FUNCTION "DIVE" : VOID
TITLE =
VERSION : 0.1


VAR_TEMP
  zero : BOOL ;
END_VAR
BEGIN
NETWORK
TITLE =Produzione in corso
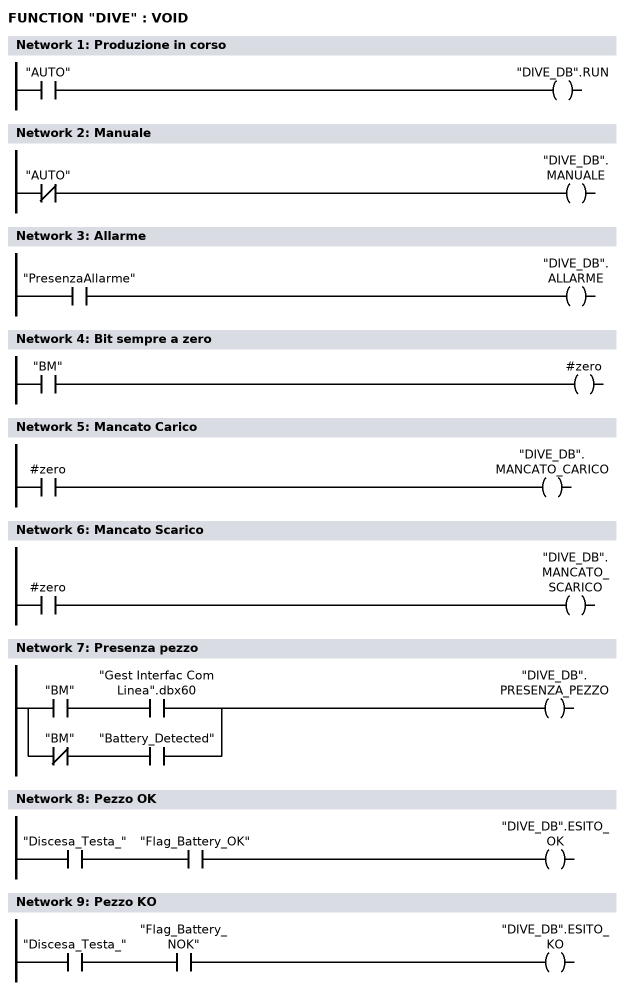
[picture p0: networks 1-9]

      U     "AUTO";
      =     "DIVE_DB".RUN;
NETWORK
TITLE =Manuale

      UN    "AUTO";
      =     "DIVE_DB".MANUALE;
NETWORK
TITLE =Allarme

      U     "PresenzaAllarme";
      =     "DIVE_DB".ALLARME;
NETWORK
TITLE =Bit sempre a zero

      U     "BM";
      =     #zero;
NETWORK
TITLE =Mancato Carico

      U     #zero;
      =     "DIVE_DB".MANCATO_CARICO;
NETWORK
TITLE =Mancato Scarico

      U     #zero;
      =     "DIVE_DB".MANCATO_SCARICO;
NETWORK
TITLE =Presenza pezzo

      U     "BM";
      U     "Gest Interfac Com Linea".dbx60;
      O     ;
      UN    "BM";
      U     "Battery_Detected";
      =     "DIVE_DB".PRESENZA_PEZZO;
NETWORK
TITLE =Pezzo OK

      U     "Discesa_Testa_";
      U     "Flag_Battery_OK";
      =     "DIVE_DB".ESITO_OK;
NETWORK
TITLE =Pezzo KO

      U     "Discesa_Testa_";
      U     "Flag_Battery_NOK";
      =     "DIVE_DB".ESITO_KO;
NETWORK
TITLE =Fine Lavoro

      U(    ;
      U     "Controllo_terminato";
      FP    M      6.4;
      S     "M6.3";
      UN    "Battery_Detected";
      R     "M6.3";
      U     "M6.3";
      )     ;
      L     S5T#500MS;
      SE    "T15";
      NOP   0;
      NOP   0;
      NOP   0;
      U     "T15";
      =     "DIVE_DB".FINE_LAVORO;
NETWORK
TITLE =Inizio Pallet
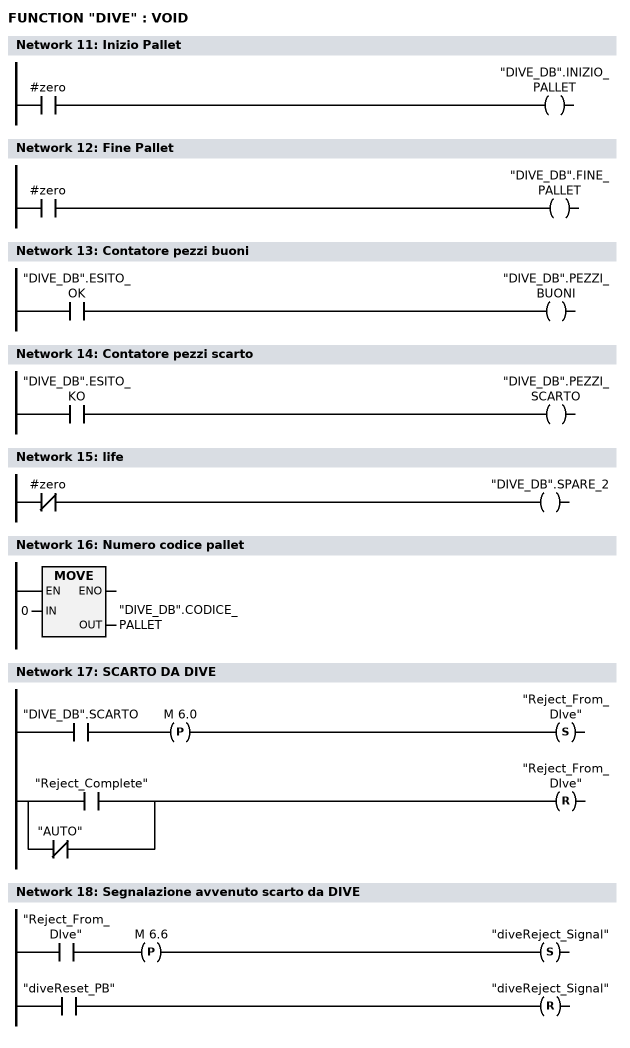
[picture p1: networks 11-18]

      U     #zero;
      =     "DIVE_DB".INIZIO_PALLET;
NETWORK
TITLE =Fine Pallet

      U     #zero;
      =     "DIVE_DB".FINE_PALLET;
NETWORK
TITLE =Contatore pezzi buoni

      U     "DIVE_DB".ESITO_OK;
      =     "DIVE_DB".PEZZI_BUONI;
NETWORK
TITLE =Contatore pezzi scarto

      U     "DIVE_DB".ESITO_KO;
      =     "DIVE_DB".PEZZI_SCARTO;
NETWORK
TITLE =life

      UN    #zero;
      =     "DIVE_DB".SPARE_2;
NETWORK
TITLE =Numero codice pallet

      L     0;
      T     "DIVE_DB".CODICE_PALLET;
      NOP   0;
NETWORK
TITLE =SCARTO DA DIVE

      U     "DIVE_DB".SCARTO;
      FP    M      6.0;
      S     "Reject_From_DIve";
      U(    ;
      O     "Reject_Complete";
      ON    "AUTO";
      )     ;
      R     "Reject_From_DIve";
      NOP   0;
NETWORK
TITLE =Segnalazione avvenuto scarto da DIVE

      U     "Reject_From_DIve";
      FP    M      6.6;
      S     "diveReject_Signal";
      U     "diveReset_PB";
      R     "diveReject_Signal";
      NOP   0;
END_FUNCTION

